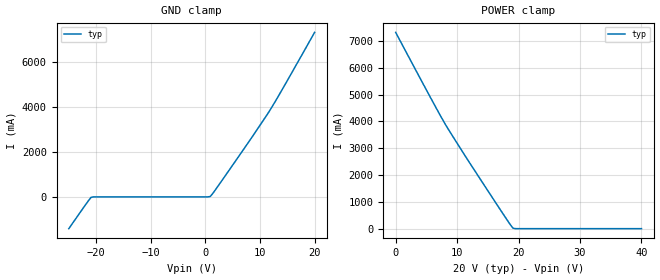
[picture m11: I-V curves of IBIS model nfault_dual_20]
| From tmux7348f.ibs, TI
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| nfault_dual_20
[Model]   nfault_dual_20
Model_type   Input
Vinl = 0.8
Vinh = 1.3
|   typ   min   max
C_comp   NA   NA
[Voltage Range]   20   NA   NA
[Temperature Range]   27   NA   NA
[Power Clamp Reference]   20   NA   NA
[GND Clamp Reference]   0   NA   NA
[GND Clamp]
|   Voltage   I(typ)   I(min)   I(max)
-25V      -1.413A    NA         NA
-20.91V   -18.23mA   NA         NA
909.1mV   18.22mA    NA         NA
6.818V    2.052A     NA         NA
11.82V    3.853A     NA         NA
14.55V    4.979A     NA         NA
20V       7.32A      NA         NA
[POWER Clamp]
|   Voltage   I(typ)   I(min)   I(max)
0V        7.32A      NA         NA
5.455V    4.979A     NA         NA
8.182V    3.853A     NA         NA
13.18V    2.052A     NA         NA
17.73V    464.3mA    NA         NA
19.09V    18.22mA    NA         NA
40V       -9.984uA   NA         NA
